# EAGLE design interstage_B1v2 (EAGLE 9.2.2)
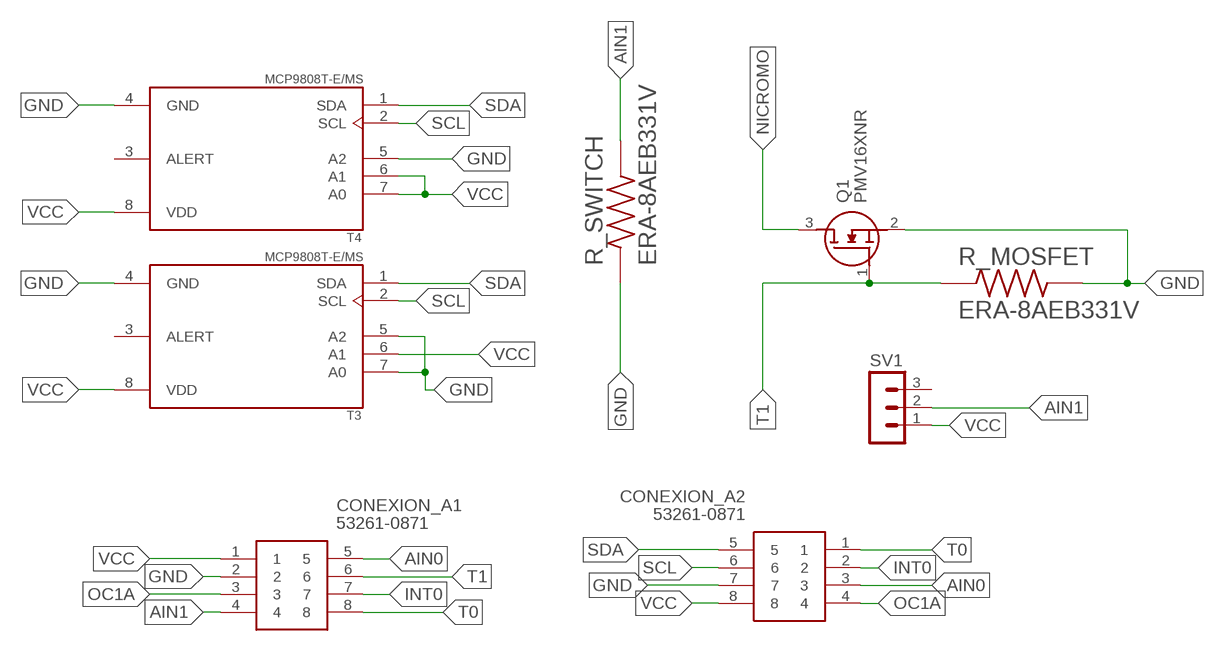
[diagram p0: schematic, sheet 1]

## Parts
CONEXION_A1  53261-0871  [53261-0871]
CONEXION_A2  53261-0871  [53261-0871]
Q1  PMV16XNR  [SOT95P230X110-3N]
R_MOSFET  ERA-8AEB331V  [RESC3216X70N]
R_SWITCH  ERA-8AEB331V  [RESC3216X70N]
SV1  MA03-1  [MA03-1]
T3  MCP9808T-E/MS  [SOP65P490X110-8N]
T4  MCP9808T-E/MS  [SOP65P490X110-8N]

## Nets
AIN0: CONEXION_A1.5 CONEXION_A2.3
AIN1: CONEXION_A1.4 R_SWITCH.2 SV1.2
GND: CONEXION_A1.2 CONEXION_A2.7 Q1.2(S) R_MOSFET.2 R_SWITCH.1 T3.4(GND) T3.5(A2) T3.7(A0) T4.4(GND) T4.5(A2)
INT0: CONEXION_A1.7 CONEXION_A2.2
NICROMO: Q1.3(D)
OC1A: CONEXION_A1.3 CONEXION_A2.4
SCL: CONEXION_A2.6 T3.2(SCL) T4.2(SCL)
SDA: CONEXION_A2.5 T3.1(SDA) T4.1(SDA)
T0: CONEXION_A1.8 CONEXION_A2.1
T1: CONEXION_A1.6 Q1.1(G) R_MOSFET.1
VCC: CONEXION_A1.1 CONEXION_A2.8 SV1.1 T3.6(A1) T3.8(VDD) T4.6(A1) T4.7(A0) T4.8(VDD)
Unconnected: SV1.3 T3.3(ALERT) T4.3(ALERT)

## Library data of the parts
CONEXION_A1 CONEXION_A2 = SamacSys_Parts:53261-0871: Molex PICOBLADE Series, Series Number 53261, 1.25mm Pitch, 8 Way 1 Row Shrouded Right Angle PCB Header, Surface Mount Source: Datasheet; DESCRIPTION: Molex PICOBLADE Series, Series Number 53261, 1.25mm Pitch, 8 Way 1 Row Shrouded Right Angle PCB Header, Surface Mount; HEIGHT: mm; MANUFACTURER_NAME: Molex; MANUFACTURER_PART_NUMBER: 53261-0871; MOUSER_PART_NUMBER: 538-53261-0871; MOUSER_PRICE-STOCK: https://www.mouser.co.uk/ProductDetail/Molex/53261-0871?qs=%252B72YyncTwW%252BggfdCJ7Netw%3D%3D
Q1 = SamacSys_Parts:PMV16XNR: Nexperia PMV16XNR N-channel MOSFET, 8.6 A, 20 V PMV16XN, 3-Pin SOT-23 Source: Datasheet; DESCRIPTION: Nexperia PMV16XNR N-channel MOSFET, 8.6 A, 20 V PMV16XN, 3-Pin SOT-23; HEIGHT: 1.1mm; MANUFACTURER_NAME: Nexperia; MANUFACTURER_PART_NUMBER: PMV16XNR; MOUSER_PART_NUMBER: 771-PMV16XNR; MOUSER_PRICE-STOCK: https://www.mouser.com/Search/Refine.aspx?Keyword=771-PMV16XNR
R_MOSFET R_SWITCH = resistor_330_smd:ERA-8AEB331V; DESCRIPTION: 330 Ohms ±0.1% 0.25W, 1/4W Chip Resistor 1206 (3216 Metric) Automotive AEC-Q200 Thin Film; DIGI-KEY_PART_NUMBER: P330BCCT-ND; MF: Panasonic Electronic; MP: ERA-8AEB331V; PACKAGE: 3216 Panasonic Electronic Components
SV1 = con-lstb:MA03-1: PIN HEADER; OC_FARNELL: unknown; OC_NEWARK: unknown
T3 T4 = sensorSPEL:MCP9808T-E/MS: Board Mount Temperature Sensors Silicon temp sensor with I2C interface; DESCRIPTION: Temperature Sensor Digital, Local -40°C ~ 125°C 10 b 8-MSOP; DIGI-KEY_PART_NUMBER: MCP9808T-E/MSCT-ND; MF: Microchip; MP: MCP9808T-E/MS; PACKAGE: MSOP-8 Microchip

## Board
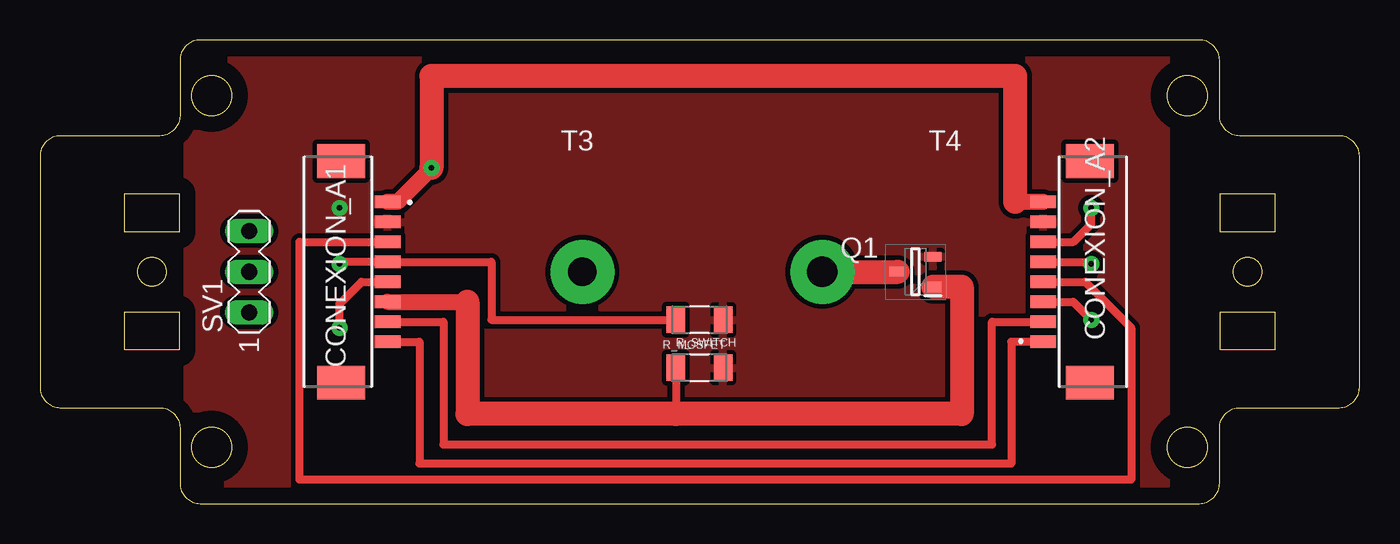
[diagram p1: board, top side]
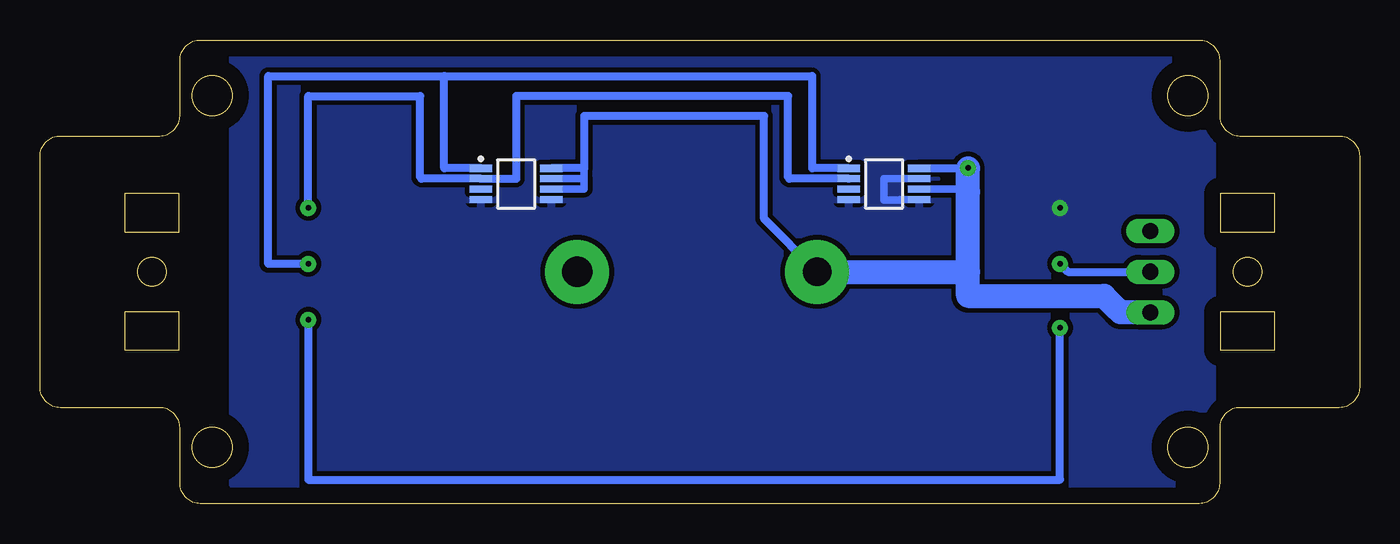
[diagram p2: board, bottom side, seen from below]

Size 82.5 x 29 mm. Coordinates in mm from the lower left corner, seen from the top.
Outline: 5.3,17 5.3,19.4 8.7,19.4 8.7,17 5.3,17
Outline: 73.8,9.6 73.8,12 77.2,12 77.2,9.6 73.8,9.6
Outline: 5.3,12 8.7,12 8.7,9.6 5.3,9.6 5.3,12
Outline: 73.8,17 73.8,19.4 77.2,19.4 77.2,17 73.8,17
Outline: 1.27,6 7.48,6 arc-90 8.75,4.73 8.75,1.27 arc90 10.02,0 72.48,0 arc90 73.75,1.27 73.75,4.73 arc-90 75.02,6 81.23,6 arc90 82.5,7.27 82.5,21.73 arc90 81.23,23 75.02,23 arc-90 73.75,24.27 73.75,27.73 arc90 72.48,29 10.02,29 arc90 8.75,27.73 8.75,24.27 arc-90 7.48,23 1.27,23 arc90 0,21.73 0,7.27 arc90 1.27,6
Outline: circle at 7,14.5 radius 0.9
Outline: circle at 75.5,14.5 radius 0.9
Outline: circle at 10.73,25.52 radius 1.25
Outline: circle at 71.72,3.52 radius 1.25
Outline: circle at 71.72,25.52 radius 1.25
Outline: circle at 10.73,3.52 radius 1.25
Copper layers (1*16): Top 0.035mm / dielectric 1.5mm / Bottom 0.035mm
Design rules "default *": minimum track width 6mil, minimum drill 0.35mm, track to track 0.3mm, track to pad 6mil, pad to pad 6mil, via to via 6mil, smd to smd 6mil, copper to edge 40mil, drill to drill 6mil, minimum pad ring 10mil, minimum via ring 8mil, stop-mask expansion 4mil, vias tented up to drill 0mil, thermal gap 10mil

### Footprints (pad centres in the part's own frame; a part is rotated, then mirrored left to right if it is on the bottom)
53261-0871 = smd 0.8 x 1.6: 1 -4.375,1.004; 2 -3.125,1.004; 3 -1.875,1.004; 4 -0.625,1.004; 5 0.625,1.004; 6 1.875,1.004; 7 3.125,1.004; 8 4.375,1.004 | smd 2.1 x 3: 9 6.925,-1.896; 10 -6.925,-1.896
SOT95P230X110-3N = smd 1.05 x 0.6: 1 -1.1,0.95; 2 -1.1,-0.95; 3 1.1,0
RESC3216X70N = smd 1.16 x 1.68: 1 -1.475,0; 2 1.475,0
MA03-1 = drill 1.016 long: 1 -2.54,0; 2 0,0; 3 2.54,0
SOP65P490X110-8N = smd 1.4 x 0.45: 1 -2.2,0.975; 2 -2.2,0.325; 3 -2.2,-0.325; 4 -2.2,-0.975; 5 2.2,-0.975; 6 2.2,-0.325; 7 2.2,0.325; 8 2.2,0.975

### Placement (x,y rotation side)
CONEXION_A1  20.73,14.5 270 top
CONEXION_A2  63.73,14.5 90 top
Q1  54.73,14.5 180 top
R_MOSFET  41.23,8.5 0 top
R_SWITCH  41.23,11.5 180 top
SV1  13.08,14.5 90 top
T3  29.73,20 0 bottom
T4  52.73,20 0 bottom

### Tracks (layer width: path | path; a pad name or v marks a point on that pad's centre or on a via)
AIN0  (via drill 0.35 pad 1)
  Top 0.5: v18.73,11 18.73,12.5 20.11,13.88 CONEXION_A1.5 | v65.73,11.5 64.61,12.62 CONEXION_A2.3
  Bottom 0.5: v65.73,11.5 65.73,1.5 18.73,1.5 v18.73,11
AIN1  (via drill 0.35 pad 1)
  Top 0.5: v18.73,15 18.73,15.12 CONEXION_A1.4 28.23,15.12 28.23,11.5 R_SWITCH.2
  Bottom 0.5: v18.73,15 18.23,14.5 SV1.2
GND  (via drill 0.35 pad 1)
  Bottom 0.47: T3.7 29.73,20.32 29.73,19 28.73,19 28.73,19.02 T3.5
  other vias: 18.73,18.5
  pour Top (isolate 0.25): 9.21,28.1 9.21,1.2 70.43,1.2 70.43,28.1
  pour Bottom (isolate 0.25): 9.23,28.1 9.23,1.2 70.43,1.2 70.43,28.1
INT0
  Top 0.5: CONEXION_A1.7 25.23,11.38 25.23,3.7 59.53,3.7 59.53,11.38 CONEXION_A2.2
NICROMO  (via drill 1.9 pad 4)
  Top 1.5: v48.91,14.5 Q1.3
OC1A
  Top 0.5: CONEXION_A1.3 16.23,16.38 16.23,1.5 68.23,1.5 68.23,11 65.36,13.88 CONEXION_A2.4
SCL  (via drill 0.35 pad 1)
  Top 0.5: CONEXION_A2.6 64.61,16.38 65.73,17.5 v65.73,18.5
  Bottom 0.5: T3.2 35.66,20.32 35.73,20.4 35.73,25.5 52.73,25.5 52.73,20.32 T4.2 58.66,20.32 58.73,20.4 58.73,25.5 65.73,25.5 v65.73,18.5
SDA  (via drill 0.35 pad 1)
  Top 0.5: CONEXION_A2.5 65.73,15.12 v65.73,15
  Bottom 0.5: T3.1 34.23,20.98 34.23,26.75 57.23,26.75 | T4.1 57.23,20.98 57.23,26.75 | v65.73,15 68.23,15 68.23,26.75 57.23,26.75
T0
  Top 0.5: CONEXION_A1.8 23.73,10.12 23.73,2.5 60.73,2.5 60.73,10.12 CONEXION_A2.1
T1
  Top 0.5: R_MOSFET.1 39.75,5.6
  Top 1: CONEXION_A1.6 26.73,12.62
  Top 1.5: Q1.1 57.63,13.55 57.63,5.6 39.75,5.6 26.73,5.6 26.73,12.62
VCC  (via drill 0.35 pad 1, 1.8 pad 4)
  Top 1: v24.48,21 22.36,18.88 CONEXION_A1.1 | CONEXION_A2.8 60.98,18.88
  Top 1.5: v24.48,21 24.48,26.75 60.98,26.75 60.98,18.88
  Bottom 0.152: 14.94,11.96 15.11,12.12
  Bottom 0.47: 24.48,19.5 24.66,19.68 T3.6 | T4.6 48.48,19.68 48.48,20.32 | 48.48,20.32 48.48,20.98 | T4.7 48.48,20.32
  Bottom 0.5: T3.8 24.48,20.98 v24.48,21 | T4.8 48.48,20.98 48.48,24.25 37.23,24.25 37.23,17.82 v33.91,14.5
  Bottom 1.5: v33.91,14.5 24.48,14.5 | 24.48,14.5 24.48,13 15.98,13 15.11,12.12 | 24.48,14.5 24.48,19.5 24.48,20.98 | SV1.1 14.94,11.96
